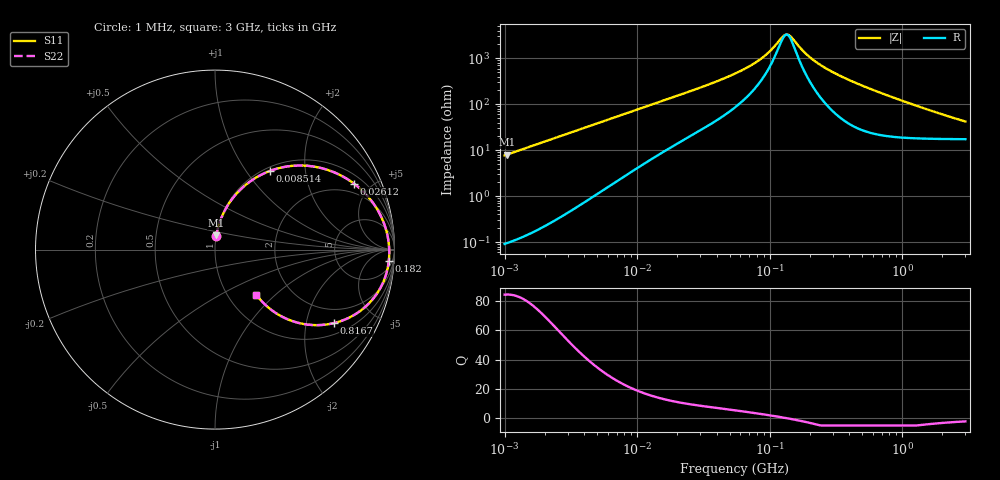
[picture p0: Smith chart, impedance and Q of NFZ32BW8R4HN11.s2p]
! NFZ32BW8R4HN11
# Hz S RI R 50
!Freq.(Hz) S11(Real) S11(Imag) S21(Real) S21(Imag) S12(Real) S12(Imag) S22(Real) S22(Imag)
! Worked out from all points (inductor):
!   401 points, 1 MHz to 3 GHz, reference 50 ohm
!   read as one part in series: L = 1.23 uH near 1.041 MHz
!   highest Q = 84.3 at 1.041 MHz (marker M1), where L = 1.23 uH
!   self-resonance near 134.1 MHz
!   S11 on the Smith chart (normalised r, x): 1 MHz: 1.00, +0.15; 8.514 MHz: 1.06, +1.31; 26.12 MHz: 1.43, +3.97; 182 MHz: 12, -25; 816.7 MHz: 1.40, -2.92; 3 GHz: 1.35, -0.77
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1000000  0.0068 0.0765  0.9932 -0.0765  0.9932 -0.0765  0.0068 0.0765
1040844  0.00732 0.0795  0.9927 -0.0795  0.9927 -0.0795  0.00732 0.0795
2055611  0.0266 0.1538  0.9734 -0.1538  0.9734 -0.1538  0.0266 0.1538
3823119  0.0849 0.2675  0.9151 -0.2675  0.9151 -0.2675  0.0849 0.2675
5705239  0.1693 0.3592  0.8307 -0.3592  0.8307 -0.3592  0.1693 0.3592
8513927  0.3073 0.4388  0.6927 -0.4388  0.6927 -0.4388  0.3073 0.4388
1.461624e7  0.5511 0.4625  0.4489 -0.4625  0.4489 -0.4625  0.5511 0.4625
2.611722e7  0.776 0.3663  0.224 -0.3663  0.224 -0.3663  0.776 0.3663
5.477226e7  0.9236 0.188  0.0764 -0.188  0.0764 -0.188  0.9236 0.188
8.679508e7  0.9591 0.0876  0.0409 -0.0876  0.0409 -0.0876  0.9591 0.0876
1.321429e8  0.9705 0.00291  0.0295 -0.00291  0.0295 -0.00291  0.9705 0.00291
1.431579e8  0.9709 -0.0133  0.0291 0.0133  0.0291 0.0133  0.9709 -0.0133
1.820241e8  0.9684 -0.0633  0.0316 0.0633  0.0316 0.0633  0.9684 -0.0633
2.094008e8  0.9639 -0.0942  0.0361 0.0942  0.0361 0.0942  0.9639 -0.0942
2.716345e8  0.9475 -0.1559  0.0525 0.1559  0.0525 0.1559  0.9475 -0.1559
3.741707e8  0.9063 -0.2392  0.0937 0.2392  0.0937 0.2392  0.9063 -0.2392
5.364635e8  0.8206 -0.333  0.1794 0.333  0.1794 0.333  0.8206 -0.333
8.005644e8  0.6726 -0.4071  0.3274 0.4071  0.3274 0.4071  0.6726 -0.4071
8.167498e8  0.6641 -0.4092  0.3359 0.4092  0.3359 0.4092  0.6641 -0.4092
1.147801e9  0.5155 -0.4178  0.4845 0.4178  0.4845 0.4178  0.5155 -0.4178
1.67892e9  0.3682 -0.3709  0.6318 0.3709  0.6318 0.3709  0.3682 -0.3709
3e9  0.2306 -0.252  0.7694 0.252  0.7694 0.252  0.2306 -0.252
